TYPE dut_GB_Input :
STRUCT

	I200_00			:BOOL;	//	PG3_LOW_ALARM
	I200_01			:BOOL;	//	PG3_HIGH_ALARM
	I200_02			:BOOL;	//	PG4_LOW_ALARM
	I200_03			:BOOL;	//	PG4_HIGH_ALARM
	I200_04			:BOOL;	//	PG5_LOW_ALARM
	I200_05			:BOOL;	//	PG5_HIGH_ALARM
	I200_06			:BOOL;	//	PG6_LOW_ALARM
	I200_07			:BOOL;	//	PG6_HIGH_ALARM
	I200_08			:BOOL;	//	PG7_LOW_ALARM
	I200_09			:BOOL;	//	PG7_HIGH_ALARM
	I200_10			:BOOL;	//	PG8_LOW_ALARM
	I200_11			:BOOL;	//	PG8_HIGH_ALARM
	I200_12			:BOOL;	//	PG31_LOW_ALARM
	I200_13			:BOOL;	//	PG31_HIGH_ALARM
	I200_14			:BOOL;	//	PG32_LOW_ALARM
	I200_15			:BOOL;	//	PG32_HIGH_ALARM
	I201_00			:BOOL;	//	LSC_H_LEVEL
	I201_01			:BOOL;	//	LSC_M_LEVEL
	I201_02			:BOOL;	//	LSC_L_LEVEL
	I201_03			:BOOL;	//	VG31_STATUS_OK
	I201_04			:BOOL;	//	VG31_LOW_ALARM
	I201_05			:BOOL;	//	VG31_HIGH_ALARM
	I201_06			:BOOL;	//	GD_FAN1_STOP
	I201_07			:BOOL;	//	GD_FAN2_STOP
	I201_08			:BOOL;	//	OX_MS1
	I201_09			:BOOL;	//	OX_MS2
	I201_10			:BOOL;	//	OX_MS3
	I201_11			:BOOL;	//	OX_MSI1
	I201_12			:BOOL;	//	OX_MSI2
	I201_13			:BOOL;	//	OX_RC1
	I201_14			:BOOL;	//	OX_RC2
	I201_15			:BOOL;	//	OX_RC3
	I202_00			:BOOL;	//	MS2_Pressure_LOW_ALARM
	I202_01			:BOOL;	//	MS2_Pressure_HIGH_ALARM
	I202_02			:BOOL;	//	MS5_Pressure_LOW_ALARM
	I202_03			:BOOL;	//	MS5_Pressure_HIGH_ALARM
	I202_04			:BOOL;	//	SPARE
	I202_05			:BOOL;	//	SPARE
	I202_06			:BOOL;	//	MP/PS20_Pressure_ALARM
	I202_07			:BOOL;	//	MP/PS11_Pressure_ALARM
	I202_08			:BOOL;	//	SPARE
	I202_09			:BOOL;	//	SPARE
	I202_10			:BOOL;	//	SPARE
	I202_11			:BOOL;	//	PG1_LOW_ALARM
	I202_12			:BOOL;	//	PG1_HIGH_ALARM
	I202_13			:BOOL;	//	SPARE
	I202_14			:BOOL;	//	SPARE
	I202_15			:BOOL;	//	SPARE
	I203_00			:BOOL;	//	SPARE
	I203_01			:BOOL;	//	SPARE	
	I203_02			:BOOL;	//	SPARE	
	I203_03			:BOOL;	//	SPARE	
	I203_04			:BOOL;	//	SPARE	
	I203_05			:BOOL;	//	SPARE	
	I203_06			:BOOL;	//	SPARE	
	I203_07			:BOOL;	//	SPARE	
	I203_08			:BOOL;	//	SPARE	
	I203_09			:BOOL;	//	SPARE	
	I203_10			:BOOL;	//	SPARE	
	I203_11			:BOOL;	//	SPARE	
	I203_12			:BOOL;	//	SPARE	
	I203_13			:BOOL;	//	SPARE	
	I203_14			:BOOL;	//	SPARE	
	I203_15			:BOOL;	//	SPARE	
	
	IW250			:INT;	//	PG3_Pressure
	IW251			:INT;	//	PG4_Pressure
	IW252			:INT;	//	PG5_Pressure
	IW253			:INT;	//	PG6_Pressure
	IW254			:INT;	//	PG7_Pressure
	IW255			:INT;	//	PG8_PressureE
	IW256			:INT;	//	PG31_Pressure
	IW257			:INT;	//	PG32_Pressure
	IW258			:INT;	//	VG31_Pressure
	IW259			:INT;	//	PG2_Pressure
	IW260			:INT;	//	PS11_Pressure
	IW261			:INT;	//	PG1_Pressure
	IW262			:INT;	//	MS2_Gasboxleft	 
	IW263			:INT;	//	MS5_Loadingarea	
	IW264			:INT;	//	OX_Value
	IW265			:INT;	//	SPARE
	IW266			:INT;	//	PG21_Pressure
	IW267			:INT;	//	PG22_Pressure
	IW268			:INT;	//	PG23_Pressure
	IW269			:INT;	//	PG33_Pressure
	
END_STRUCT
END_TYPE
